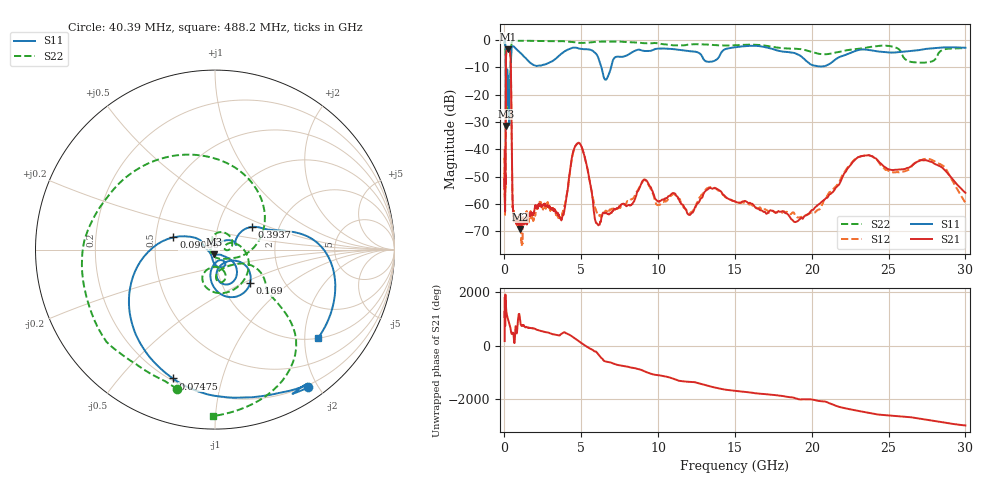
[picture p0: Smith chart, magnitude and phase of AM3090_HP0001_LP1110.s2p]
! Date/Time: Thu, Feb 28, 2019 1:54 PM
! Network Analyzer: Agilent Technologies E8364B Rev: A.07.50.67
! Sweep from 0.010 to 30.000 GHz, 1601 Points, Sweep Type: LOG
! Power Supply: 5.022 V, 0.002 A
# Hz S DB R 50
!freq MagS11 AngS11 MagS21 AngS21 MagS12 AngS12 MagS22 AngS22
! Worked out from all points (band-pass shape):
!   1601 points, 10 MHz to 30 GHz, reference 50 ohm
!   highest |S21| = -3.43 dB at 256 MHz (marker M1); lowest = -69.1 dB at 988.5 MHz (marker M2)
!   |S21| within 3 dB of the highest: 101.5 MHz to 396.6 MHz (295.1 MHz wide, 119 % of centre)
!   lowest |S11| = -31.5 dB at 98.93 MHz (marker M3), VSWR 1.05, Z = 49.5 - j2.61 ohm
!   |S11| at or under -10 dB: 89.63 MHz to 409 MHz (319.4 MHz wide, 128 % of centre); 6.31 GHz to 6.936 GHz (626.6 MHz wide, 9.46 % of centre)
!   |S22| runs from -32.8 to -0.2 dB; largest |S21 - S12| = 0.013
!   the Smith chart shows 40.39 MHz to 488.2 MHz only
!   S11 on the Smith chart (normalised r, x): 40.39 MHz: 0.17, -1.87; 74.75 MHz: 0.21, -0.70; 90.86 MHz: 0.62, +0.09; 169 MHz: 1.36, -0.54; 393.7 MHz: 1.45, +0.39; 488.2 MHz: 1.00, -2.32
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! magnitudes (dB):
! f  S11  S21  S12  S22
! 10 MHz  -0.2  -40.2  -43.9  -0.7
! 38.04 MHz  -0.5  -62.5  -62.3  -1.7
! 40.39 MHz  -0.7  -62.6  -60.0  -1.9
! 74.75 MHz  -2.4  -48.3  -45.7  -4.3
! 90.86 MHz  -12.3  -14.2  -14.1  -13.2
! 98.93 MHz  -31.5  -7.2  -7.2  -32.6
! 144.7 MHz  -19.0  -3.6  -3.6  -24.2
! 169 MHz  -11.4  -3.5  -3.5  -14.3
! 256 MHz  -22.0  -3.4  -3.4  -17.9
! 312.7 MHz  -31.0  -3.8  -3.8  -16.1
! 393.7 MHz  -12.4  -6.2  -6.2  -10.3
! 488.2 MHz  -2.4  -44.7  -44.6  -0.7
! 550.5 MHz  -2.3  -61.1  -62.0  -0.4
! 988.5 MHz  -4.5  -69.1  -64.8  -0.3
! 2.084 GHz  -9.5  -60.5  -60.9  -0.3
! 3.742 GHz  -4.9  -65.4  -64.1  -0.4
! 4.805 GHz  -3.1  -37.7  -37.6  -1.0
! 6.049 GHz  -5.8  -67.3  -63.7  -0.7
! 7.926 GHz  -5.8  -60.8  -59.8  -0.8
! 19.22 GHz  -5.6  -65.5  -64.9  -3.3
! 23.48 GHz  -3.5  -42.2  -42.2  -2.9
! 30 GHz  -2.9  -55.9  -59.5  -3.0
